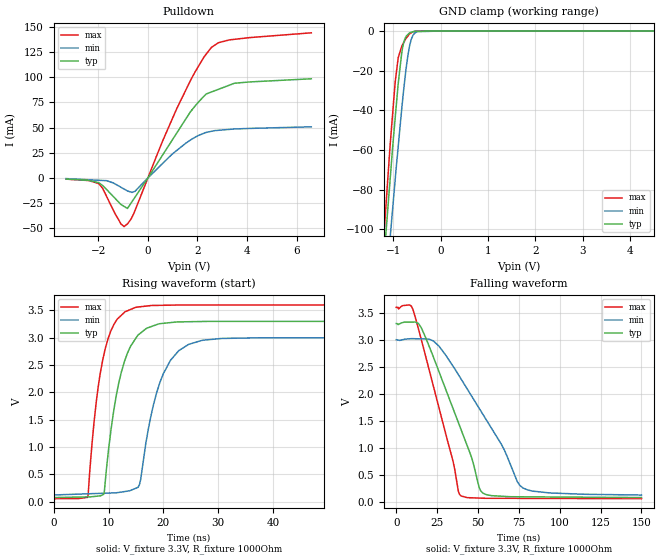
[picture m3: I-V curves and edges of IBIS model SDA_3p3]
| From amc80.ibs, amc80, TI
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|   SDA model
[Model]  SDA_3p3
Model_type   I/O_open_drain
Polarity   Non-Inverting
Enable   Active-Low
Vinl = 0.8
Vinh = 2
Vmeas = 1.65
Vref = 1.65
Cref = 15pF
Rref = 50
|   typ   min   max
|   (nom PVT)   (Fast PVT)   (slow PVT)
|   BUFFER OUTPUT TURNED HIGH or as an INPUT
|C_comp   1.340E-12   1.028E-12   1.479E-12
|   BUFFER OUTPUT TURNED LOW
C_comp   8.997E-13   8.832E-13   9.819E-13
| Where   nom PVT is  Nominal Process, 3.3V, 27C
|   Fast PVT is Strong Process, 3.6V, -40C
|   Slow PVT is Weak Process, 3.0V, 125C
|C_comp - from L-C Tank method, L = 1nH, peak frequency
[Voltage Range]   3.3   3   3.6
[Temperature Range]   27   125   -40
[Pullup Reference]   3.3   3   3.6
[Pulldown Reference]   0   0   0
[Power Clamp Reference]   3.3   3   3.6
[GND Clamp Reference]   0   0   0
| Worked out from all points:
|   slope of the pulldown table from 0 to 0.495 V, typ, clamps not added: 26.1 ohm
|   GND clamp passes 1 mA (typ) near -0.66 V on its own axis
|   falling waveform, V_fixture 3.3V, R_fixture 1000Ohm: 20-80 % time 24ns typ, 33.1ns min, 18.3ns max; typ from 3.3 V to 0.077 V
|   rising waveform, V_fixture 3.3V, R_fixture 1000Ohm: 20-80 % time 3.48ns typ, 4.16ns min, 2.91ns max; typ from 0.077 V to 3.3 V
[Pulldown]
|   Voltage   I(typ)   I(min)   I(max)
-3.3V     -1.175mA   -709.3uA   -1.236mA
-1.971V   -4.981mA   -2.394mA   -5.901mA
-1.086V   -26.42mA   -9.342mA   -45.79mA
-960.8mV  -28.34mA   -11.1mA    -48.44mA
-826.2mV  -30.42mA   -12.99mA   -45.81mA
-522.4mV  -19.23mA   -13.36mA   -32.57mA
1.169V    44.82mA    27.42mA    69.19mA
1.894V    71.22mA    40.31mA    105mA
2.356V    83.5mA     45.27mA    123.3mA
2.556V    85.38mA    46.3mA     129.7mA
3.491V    94.14mA    48.64mA    137.8mA
6.59V     98.58mA    50.8mA     144.3mA
[GND Clamp]
|   Voltage   I(typ)   I(min)   I(max)
-3.3V     -813.1mA   -775.3mA   -896.6mA
-1.229V   -123.9mA   -150.1mA   -112.5mA
-1.179V   -107.9mA   -135.4mA   -95.05mA
-1.109V   -86.53mA   -115mA     -70.83mA
-1.072V   -75.38mA   -104.9mA   -58.16mA
-1.019V   -59.07mA   -90.13mA   -42.1mA
-969.9mV  -45.57mA   -76.63mA   -27.41mA
-899.8mV  -26.56mA   -58.26mA   -13.44mA
-785.8mV  -6.001mA   -30.03mA   -5.896mA
-660.9mV  -914.2uA   -7.649mA   -1.498mA
-500.7mV  -89.74uA   -329.2uA   -49.27uA
6.59V     0A         0A         0A
[POWER Clamp]
|   SCR cell for ESD function. Effects occurr above VDD x 2
|   Voltage   I(typ)   I(min)   I(max)
-3.3V     0A         0A         0A
0V        0A         0A         0A
6.6V      0A         0A         0A
[Ramp]
R_load = 1000
|   typ   min   max
dV/dt_r   1.93406/3.46886e-009   1.7257/4.10542e-009   2.12641/2.90654e-009
dV/dt_f   1.93406/2.39881e-008   1.72582/3.31486e-008   2.12641/1.83051e-008
[Falling Waveform]
V_fixture = 3.3V
V_fixture_min = 3V
V_fixture_max = 3.6V
R_fixture = 1000Ohm
C_fixture = 0F
|   Time   V(typ)   V(min)   V(max)
0s        3.3V       3V         3.6V
10.23ns   3.328V     3.02V      3.558V
15.3ns    3.221V     3.016V     3.005V
22.76ns   2.676V     2.977V     2.133V
38.05ns   1.461V     2.351V     187.9mV
39.41ns   1.353V     2.284V     111mV
46.29ns   798mV      1.947V     72.21mV
51.66ns   200.5mV    1.683V     66.21mV
77.21ns   91.11mV    261.2mV    61.77mV
150ns     76.57mV    123.6mV    55.99mV
[Rising Waveform]
V_fixture = 3.3V
V_fixture_min = 3V
V_fixture_max = 3.6V
R_fixture = 1000Ohm
C_fixture = 0F
|   Time   V(typ)   V(min)   V(max)
0s        76.57mV    123.8mV    55.99mV
6.183ns   88.97mV    145.3mV    81.36mV
7.706ns   100.3mV    150.6mV    1.794V
9.09ns    138.8mV    155.4mV    2.669V
11.85ns   2.175V     170.6mV    3.366V
14.87ns   2.976V     243.3mV    3.553V
15.62ns   3.07V      312.2mV    3.565V
19.97ns   3.264V     2.341V     3.593V
26.94ns   3.297V     2.949V     3.599V
150ns     3.3V       3V         3.6V
